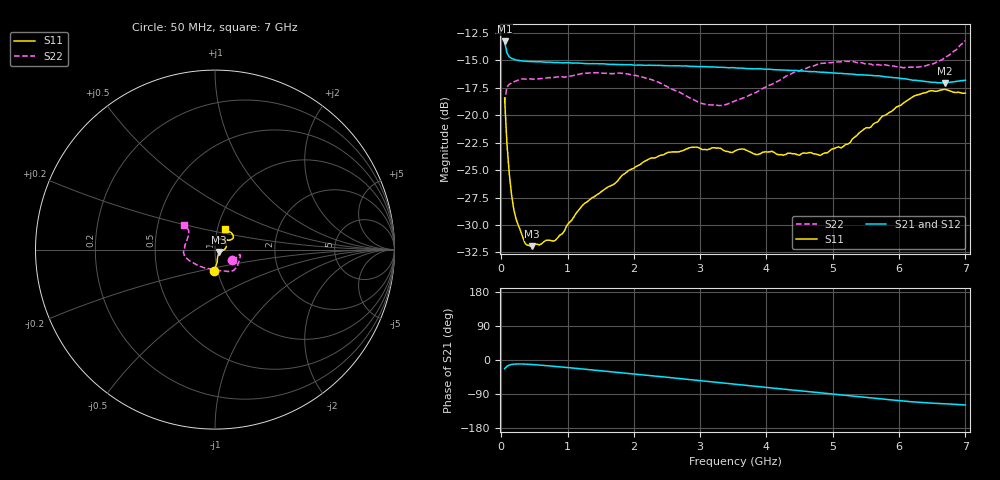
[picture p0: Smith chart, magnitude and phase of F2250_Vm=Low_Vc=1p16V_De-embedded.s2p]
! Integrated Device Technology
! Corporate Headquarters
! 6024 Silver Creek Valley Road
! San Jose, CA 95138  USA
! Phone:  1-408-284-8200
! Toll Free:  1-800-223-1366
! Webpage:  http://www.idt.com/
! Timing and RF Division
! 515 Groton Road, Suite 102
! Westford, MA 01886-6024
! Device:  F2250
! Description: Voltage Variable RF Attenuator
! Frequency:  50.0 -  6000.00 MHz
! Package:  3x3 mm Thin QFN Plastic Package: 16 pin
! Ports:  2 RF, 3 DC
!  Pin  1  = GND
!  Pin  2  = NC
!  Pin  3  = RF1  = Port 1
!  Pin  4  = NC
!  Pin  5  = GND
!  Pin  6  = GND
!  Pin  7  = GND
!  Pin  8  = GND
!  Pin  9  = NC
!  Pin 10  = RF2  = Port 2
!  Pin 11  = NC
!  Pin 12  = GND
!  Pin 13  = GND
!  Pin 14  = VCNTRL
!  Pin 15  = VDD
!  Pin 16  = VMODE
! Vcntrl:  1.160 Volts
! Vmode:  +0.000 Volts
! Vdd:  +3.30  Volts
! Current:  1.193 mA
! Data:  The device was measured on a the F2250 evaluation board which has
!  individual transmission lines to the RF pins.  Data was collected
!  using a calibrated network analyzer.  The evaluation board was
!  de-embedded using a TRL calibration technique.
!  The reference plane is the edge of the package pin.
! Misc:  SN 10
!  Action Tracker AT0258
! Date Measured:  2014-11-26
! Date:  2015-10-15  MJV
! Note:
!  Integrated Device Technology supplies this data as a sample of measured
!  data at the package pin for this product.  Your particular data for this
!  product may vary.
!  Data was taken at 25 degrees C.
!  Integrated Device Technology reserves the right to change this data at anytime.
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# GHz S dB R 50
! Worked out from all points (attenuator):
!   201 points, 50 MHz to 7 GHz, reference 50 ohm
!   highest |S21| = -13.28 dB at 50 MHz (marker M1); lowest = -17.1 dB at 6.687 GHz (marker M2)
!   lowest |S11| = -31.9 dB at 467 MHz (marker M3), VSWR 1.05, Z = 52.2 - j1.43 ohm
!   |S11| at or under -10 dB: start of sweep to end of sweep
!   |S22| runs from -19.1 to -13.2 dB; largest |S21 - S12| = 0.00061
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0.05  -18.42 -92.7  -13.28 -23.1  -13.27 -23.0  -18.85 -31.8
0.08475  -22.55 -81.2  -14.32 -16.7  -14.32 -16.7  -17.43 -16.5
0.1195  -25.27 -75.5  -14.68 -13.5  -14.68 -13.5  -17.19 -12.5
0.15425  -27.23 -70.2  -14.82 -11.9  -14.83 -11.9  -17.07 -11.4
0.189  -28.61 -63.2  -14.90 -11.0  -14.91 -11.0  -16.95 -11.3
0.36275  -31.72 -39.4  -15.08 -10.9  -15.08 -10.9  -16.71 -13.4
0.467  -31.93 -32.7  -15.12 -11.9  -15.11 -11.9  -16.71 -15.7
0.8145  -31.40 -18.1  -15.20 -16.9  -15.21 -16.9  -16.54 -25.9
1.2315  -28.17 -12.2  -15.28 -23.8  -15.27 -23.8  -16.18 -36.5
1.9265  -25.01 4.8  -15.39 -35.6  -15.38 -35.6  -16.27 -49.8
2.37825  -23.70 15.9  -15.46 -43.4  -15.47 -43.4  -17.01 -59.8
2.86475  -22.93 31.5  -15.56 -52.1  -15.55 -52.1  -18.48 -78.1
3.0385  -23.13 37.9  -15.57 -55.2  -15.56 -55.2  -18.95 -87.4
3.3165  -23.04 48.0  -15.63 -60.2  -15.63 -60.2  -19.11 -105.0
3.525  -23.25 53.5  -15.68 -63.9  -15.68 -63.9  -18.69 -118.0
4.7065  -23.51 63.8  -16.02 -85.0  -16.03 -85.0  -15.51 -164.1
4.81075  -23.67 60.0  -16.08 -86.8  -16.05 -86.9  -15.28 -166.0
5.1235  -22.97 50.2  -16.18 -92.4  -16.18 -92.4  -15.14 -172.8
5.85325  -19.74 31.9  -16.54 -104.9  -16.53 -104.9  -15.49 170.7
6.2355  -18.22 33.2  -16.81 -110.8  -16.81 -110.8  -15.64 158.0
6.68725  -17.65 45.7  -17.06 -115.5  -17.05 -115.5  -14.74 143.7
7  -17.99 64.1  -16.80 -118.8  -16.82 -118.8  -13.19 142.2
